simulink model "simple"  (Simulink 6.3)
settings: Solver=ode45  StartTime=0.0  StopTime=25.0  RelTol=1e-3
undefined symbols (not defined in the file or in its folder): Bit, Location, Lower, netlist, Width
libraries: xbsIndex_r4 x17, adlibrary2 x1

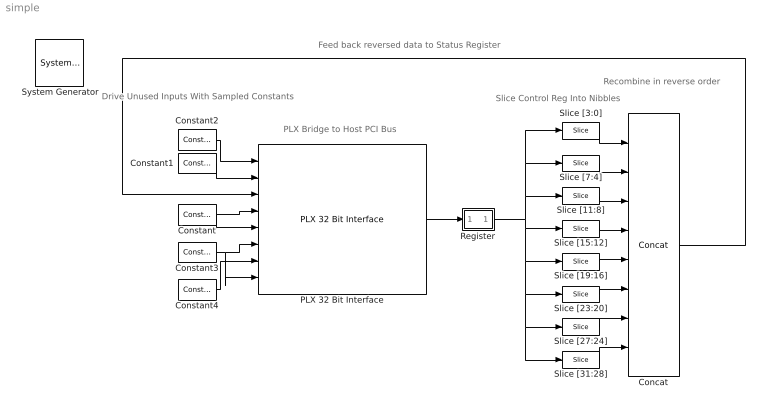
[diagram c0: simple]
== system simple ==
  note: Drive Unused Inputs With Sampled Constants
  note: PLX Bridge to Host PCI Bus
  note: Slice Control Reg Into Nibbles
  note: Recombine in reverse order
  note: Feed back reversed data to Status Register
  " System Generator" : xbsIndex_r4/ System Generator  Tag=genX  xilinxfamily=Virtex4  part=xc4vsx55  speed=-10  package=ff1148  synthesis_tool=XST  directory=./netlist  testbench=off  simulink_period=1  sysclk_period=7.5  incr_netlist=off  trim_vbits=Everywhere in SubSystem  dbl_ovrd=According to Block Masks  core_generation=According to Block Masks  run_coregen=off  deprecated_control=off  eval_field=0  block_type=sysgen
  Concat : xbsIndex_r4/Concat  num_inputs=8  dbl_ovrd=off  block_type=concat
  Constant : xbsIndex_r4/Constant  arith_type=Boolean  const=0  n_bits=1  bin_pt=0  explicit_period=on  period=1  equ=P=C  opselect=C  inp2=PCIN>>17  opr=+  inp1=P  carry=CIN  dbl_ovrd=off  block_type=constant
  Constant1 : xbsIndex_r4/Constant  arith_type=Boolean  const=1  n_bits=1  bin_pt=0  explicit_period=on  period=1  equ=P=C  opselect=C  inp2=PCIN>>17  opr=+  inp1=P  carry=CIN  dbl_ovrd=off  block_type=constant
  Constant2 : xbsIndex_r4/Constant  arith_type=Unsigned  const=0  n_bits=32  bin_pt=0  explicit_period=on  period=1  equ=P=C  opselect=C  inp2=PCIN>>17  opr=+  inp1=P  carry=CIN  dbl_ovrd=off  block_type=constant
  Constant3 : xbsIndex_r4/Constant  arith_type=Unsigned  const=0  n_bits=32  bin_pt=0  explicit_period=on  period=1  equ=P=C  opselect=C  inp2=PCIN>>17  opr=+  inp1=P  carry=CIN  dbl_ovrd=off  block_type=constant
  Constant4 : xbsIndex_r4/Constant  arith_type=Unsigned  const=0  n_bits=34  bin_pt=0  explicit_period=on  period=1  equ=P=C  opselect=C  inp2=PCIN>>17  opr=+  inp1=P  carry=CIN  dbl_ovrd=off  block_type=constant
  PLX 32 Bit Interface : adlibrary2/ADM-XRC-II/PLX 32 Bit Interface  program='slave_write 0x40000 0x1bcd1234;slave_read 0x40040'  clock_ratio=1.5
  Register : Subsystem
  Slice [11:8] : xbsIndex_r4/Slice  nbits=4  boolean_output=off  mode=Lower Bit Location + Width  bit1=0  base1=MSB of Input  bit0=8  base0=LSB of Input  dbl_ovrd=off  block_type=slice
  Slice [15:12] : xbsIndex_r4/Slice  nbits=4  boolean_output=off  mode=Lower Bit Location + Width  bit1=0  base1=MSB of Input  bit0=12  base0=LSB of Input  dbl_ovrd=off  block_type=slice
  Slice [19:16] : xbsIndex_r4/Slice  nbits=4  boolean_output=off  mode=Lower Bit Location + Width  bit1=0  base1=MSB of Input  bit0=16  base0=LSB of Input  dbl_ovrd=off  block_type=slice
  Slice [23:20] : xbsIndex_r4/Slice  nbits=4  boolean_output=off  mode=Lower Bit Location + Width  bit1=0  base1=MSB of Input  bit0=20  base0=LSB of Input  dbl_ovrd=off  block_type=slice
  Slice [27:24] : xbsIndex_r4/Slice  nbits=4  boolean_output=off  mode=Lower Bit Location + Width  bit1=0  base1=MSB of Input  bit0=24  base0=LSB of Input  dbl_ovrd=off  block_type=slice
  Slice [31:28] : xbsIndex_r4/Slice  nbits=4  boolean_output=off  mode=Lower Bit Location + Width  bit1=0  base1=MSB of Input  bit0=28  base0=LSB of Input  dbl_ovrd=off  block_type=slice
  Slice [3:0] : xbsIndex_r4/Slice  nbits=4  boolean_output=off  mode=Lower Bit Location + Width  bit1=0  base1=MSB of Input  bit0=0  base0=LSB of Input  dbl_ovrd=off  block_type=slice
  Slice [7:4] : xbsIndex_r4/Slice  nbits=4  boolean_output=off  mode=Lower Bit Location + Width  bit1=0  base1=MSB of Input  bit0=4  base0=LSB of Input  dbl_ovrd=off  block_type=slice
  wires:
  Constant/1 -> PLX 32 Bit Interface/4, PLX 32 Bit Interface/5
  Constant1/1 -> PLX 32 Bit Interface/2
  Constant2/1 -> PLX 32 Bit Interface/1
  Constant3/1 -> PLX 32 Bit Interface/6, PLX 32 Bit Interface/8
  Constant4/1 -> PLX 32 Bit Interface/7
  PLX 32 Bit Interface/6 -> Register/1(in0)
  Register/1(out0) -> Slice [31:28]/1, Slice [27:24]/1, Slice [23:20]/1, Slice [19:16]/1, Slice [15:12]/1, Slice [11:8]/1, Slice [3:0]/1, Slice [7:4]/1
  Slice [3:0]/1 -> Concat/1
  Slice [7:4]/1 -> Concat/2
  Slice [11:8]/1 -> Concat/3
  Slice [15:12]/1 -> Concat/4
  Slice [19:16]/1 -> Concat/5
  Slice [23:20]/1 -> Concat/6
  Slice [27:24]/1 -> Concat/7
  Slice [31:28]/1 -> Concat/8
  Concat/1 -> PLX 32 Bit Interface/3

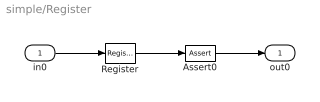
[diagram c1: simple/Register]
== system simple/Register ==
  in0 : Inport
  Assert0 : xbsIndex_r4/Assert  assert_type=off  type_source=Explicitly  arith_type="Signed  (2's comp)"  n_bits=16  bin_pt=14  assert_rate=on  rate_source=Explicitly  period=1  output_port=on  block_type=assert
  Register : xbsIndex_r4/Register  init=0  rst=off  en=off  dbl_ovrd=off  block_type=register
  out0 : Outport
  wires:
  in0/1 -> Register/1
  Register/1 -> Assert0/1
  Assert0/1 -> out0/1
